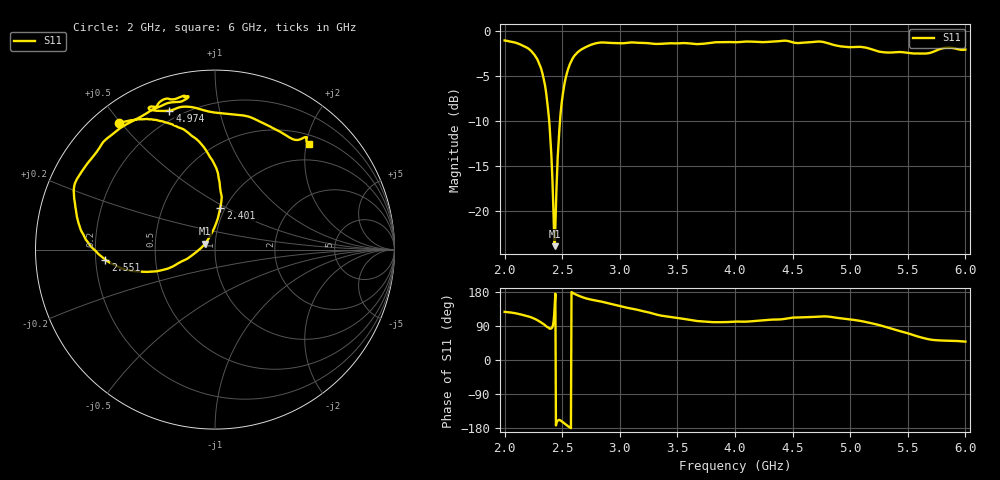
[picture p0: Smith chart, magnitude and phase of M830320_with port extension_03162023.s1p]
# Hz S RI R 50
! CMT, M5090, 19127454, 21.2.4/2
! Date: 3/16/2023 5:09:15 PM
! Data: Format (Calibration Info)
! Freq	S11:Re/Im(F2 Pxt)
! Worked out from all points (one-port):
!   800 points, 2 GHz to 6 GHz, reference 50 ohm
!   lowest |S11| = -24.0 dB at 2.436 GHz (marker M1), VSWR 1.14, Z = 44.8 + j2.98 ohm
!   |S11| at or under -10 dB: 2.387 GHz to 2.481 GHz (93.84 MHz wide, 3.86 % of centre)
!   S11 on the Smith chart (normalised r, x): 2 GHz: 0.07, +0.50; 2.401 GHz: 0.95, +0.46; 2.551 GHz: 0.24, -0.04; 4.974 GHz: 0.16, +0.71; 6 GHz: 0.66, +2.05
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2e9  -0.5343 0.7074
2.180225e9  -0.3716 0.7263
2.295369e9  -0.1505 0.6521
2.360451e9  0.00711 0.4539
2.380476e9  0.0278 0.3486
2.400501e9  0.0292 0.2313
2.420526e9  -0.00545 0.1172
2.435544e9  -0.0541 0.0331
2.450563e9  -0.1302 -0.0337
2.475594e9  -0.2638 -0.1062
2.500626e9  -0.4058 -0.1233
2.550688e9  -0.6106 -0.056
2.620776e9  -0.7411 0.0964
2.730914e9  -0.7826 0.2735
2.841051e9  -0.7763 0.3783
3.001252e9  -0.6766 0.5215
3.326658e9  -0.4134 0.7404
3.501877e9  -0.3064 0.7973
3.782228e9  -0.1524 0.8446
4.002503e9  -0.1712 0.8496
4.503129e9  -0.3222 0.8029
4.773467e9  -0.3688 0.7849
4.973717e9  -0.2536 0.7738
5.003755e9  -0.2376 0.778
5.198999e9  -0.0834 0.7826
5.50438e9  0.2575 0.7097
5.744681e9  0.4766 0.615
6e9  0.5221 0.5908
